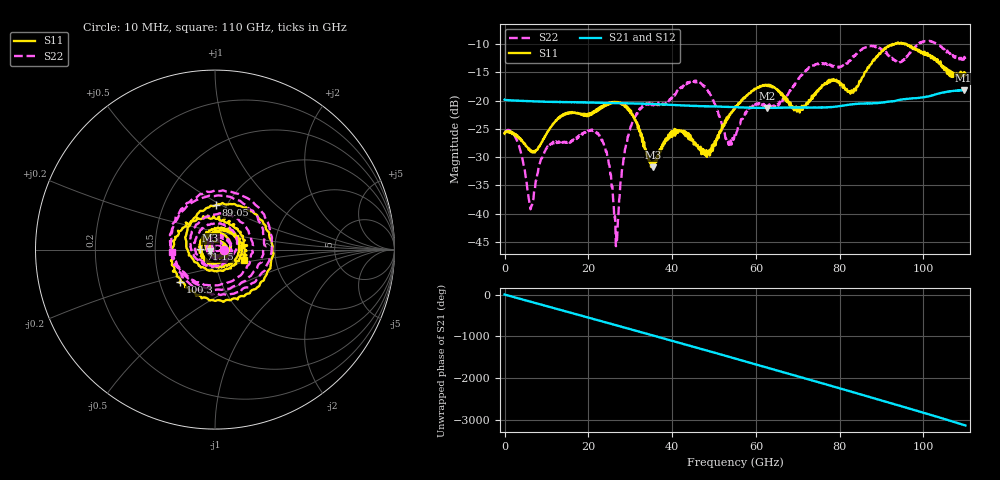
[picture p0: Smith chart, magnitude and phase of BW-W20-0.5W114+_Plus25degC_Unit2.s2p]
!Mini-Circuits Laboratory
!S-Parameters
!Model: BW-W20-0.5W114+
!Run / Lot / Date Code: QN2409253 /  / N/A
!Fixture:
!Network Analyzer: PNA-X N5242B - 423 4 ports (COM/DCOM);  Serial number: 74408
!Date: 3/8/2024 at 1:33:02 PM
!No.: Unit# 5 (U2  25C)
!Tested with:
# Hz  S  dB  R  50
!Frequency  S11 dB  S11 Deg  S21 dB  S21 Deg  S12 dB  S12 Deg  S22 dB  S22 Deg
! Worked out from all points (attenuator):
!   2208 points, 10 MHz to 110 GHz, reference 50 ohm
!   highest |S21| = -18.15 dB at 109.5 GHz (marker M1); lowest = -21.3 dB at 62.75 GHz (marker M2)
!   lowest |S11| = -31.8 dB at 35.55 GHz (marker M3), VSWR 1.05, Z = 47.6 - j0.499 ohm
!   |S11| at or under -10 dB: start of sweep to 92.6 GHz; 92.68995 GHz to 93.11505 GHz (425.1 MHz wide, 0.458 % of centre); 95.87 GHz to end of sweep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
!   |S22| runs from -45.8 to -9.4 dB; largest |S21 - S12| = 0.0065
!   S11 on the Smith chart (normalised r, x): 10 MHz: 1.11, +0.00; 71.15 GHz: 0.85, +0.01; 89.05 GHz: 0.90, +0.47; 100.3 GHz: 0.64, -0.25; 110 GHz: 1.37, -0.16
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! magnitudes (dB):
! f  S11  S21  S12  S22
! 10 MHz  -25.9  -19.8  -19.8  -25.8
! 3.2 GHz  -26.6  -20.0  -20.0  -27.6
! 6.35 GHz  -28.8  -20.1  -20.1  -38.7
! 10.05 GHz  -25.9  -20.2  -20.2  -28.5
! 18.35 GHz  -22.5  -20.3  -20.3  -26.1
! 23.85 GHz  -21.0  -20.4  -20.4  -28.2
! 26.65 GHz  -20.4  -20.4  -20.4  -44.6
! 29.9 GHz  -21.7  -20.5  -20.5  -25.2
! 35.55 GHz  -31.8  -20.6  -20.6  -20.8
! 36.7 GHz  -29.5  -20.7  -20.6  -20.4
! 41.35 GHz  -25.7  -20.8  -20.8  -18.4
! 46.2 GHz  -28.3  -21.0  -21.0  -16.9
! 55.05 GHz  -21.1  -21.2  -21.1  -25.9
! 62.75 GHz  -17.2  -21.3  -21.3  -21.0
! 71.15 GHz  -21.6  -21.2  -21.2  -15.2
! 73.35 GHz  -19.1  -21.2  -21.2  -13.8
! 83.4 GHz  -18.0  -20.6  -20.7  -12.2
! 89.05 GHz  -12.1  -20.4  -20.3  -10.5
! 91.7 GHz  -10.5  -20.2  -20.0  -12.1
! 100.3 GHz  -11.5  -19.4  -19.3  -9.5
! 109.5 GHz  -15.0  -18.2  -18.0  -12.8
! 110 GHz  -15.4  -18.2  -18.0  -12.4
